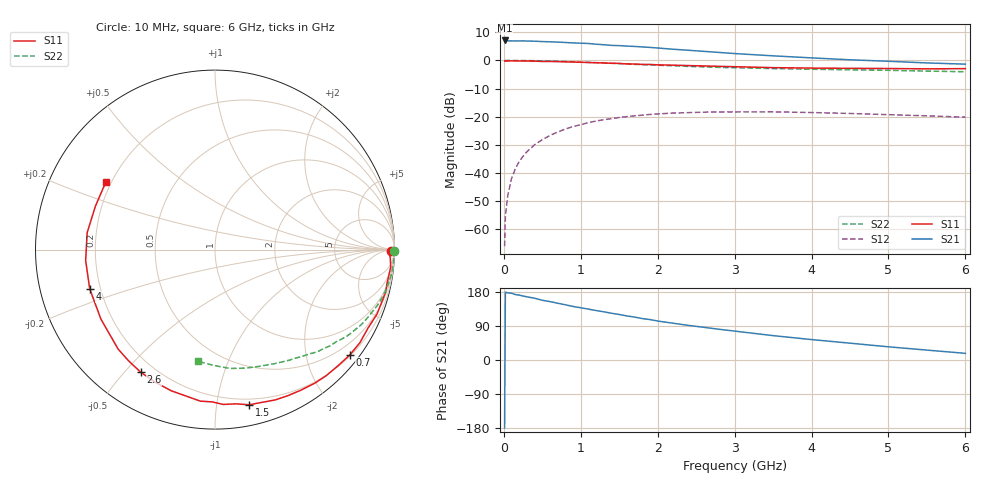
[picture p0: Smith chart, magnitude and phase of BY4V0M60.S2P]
! SIEMENS Small Signal Semiconductors
! BFY420
! Si NPN RF SIEGET Grounded Emitter Transistor in MICRO-X
! VCE = 4 V  IC = 0.6 mA
! Common Emitter S-Parameters:  October  1996
# GHz  S  MA  R  50
!  f  S11  S21  S12  S22
! GHz  MAG  ANG  MAG  ANG  MAG  ANG  MAG  ANG
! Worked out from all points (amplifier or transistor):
!   36 points, 10 MHz to 6 GHz, reference 50 ohm
!   highest |S21| = 7.1 dB at 10 MHz (marker M1)
!   |S21| within 3 dB of that: start of sweep to 2.146 GHz
!   unconditionally stable (mu >= 1): 4.683 GHz to end of sweep
!   at 250 MHz: K = 0.04, MSG = 20.5 dB, |S12| = -34.1 dB
!   at 1.4 GHz: K = 0.16, MSG = 13.0 dB, |S12| = -20.7 dB
!   at 6 GHz: K = 1.43, MAG = 5.5 dB, |S12| = -20.2 dB
!   S11 on the Smith chart (normalised r, x): 10 MHz: 78, -41; 700 MHz: 0.22, -2.89; 1.5 GHz: 0.15, -1.23; 2.6 GHz: 0.15, -0.55; 4 GHz: 0.16, -0.15; 6 GHz: 0.18, +0.27
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0.01  0.9802 -0.6  2.265 -179.3  0.0005 88.5  0.9999 -0.3
0.02  0.97 -1.3  2.243 178.9  0.0017 96.1  0.9955 -0.4
0.05  0.9777 -2.6  2.228 177.3  0.0039 85.0  0.9985 -1.2
0.1  0.9836 -5.6  2.228 176.1  0.008 84.7  0.996 -2.5
0.15  0.9794 -8.4  2.215 172.7  0.0119 83.4  0.9972 -3.7
0.25  0.9793 -13.7  2.227 168.9  0.0198 80.9  0.9948 -6.0
0.4  0.9715 -21.7  2.199 163.1  0.0318 76.6  0.988 -9.8
0.5  0.9579 -27.3  2.164 157.6  0.039 73.1  0.9816 -12.2
0.7  0.9532 -38.0  2.118 149.8  0.0534 66.8  0.9658 -16.8
0.9  0.9367 -48.7  2.05 141.3  0.0669 60.2  0.9444 -21.2
1.1  0.9179 -58.6  2 134.2  0.0787 54.3  0.924 -25.6
1.5  0.885 -77.6  1.834 120.1  0.0967 42.8  0.8785 -33.3
1.8  0.8486 -91.1  1.738 109.3  0.1066 35.7  0.843 -38.4
2.2  0.8235 -107.2  1.582 97.1  0.116 26.8  0.8062 -44.9
2.6  0.7988 -121.2  1.45 86.3  0.1203 19.5  0.7689 -50.6
3  0.7738 -134.2  1.325 76.3  0.1218 13.1  0.7424 -56.1
3.5  0.7442 -148.7  1.207 64.3  0.122 6.8  0.7173 -62.3
4  0.7315 -162.6  1.11 53.9  0.1186 1.8  0.697 -68.7
4.5  0.7232 -175.2  1.027 44.4  0.1141 -2.2  0.6826 -75.3
5  0.7184 172.4  0.966 34.8  0.1087 -4.6  0.6677 -82.7
5.5  0.7088 160.0  0.903 26.1  0.1035 -5.3  0.6464 -90.2
6  0.715 148.4  0.859 17.6  0.0981 -4.2  0.6296 -98.6
